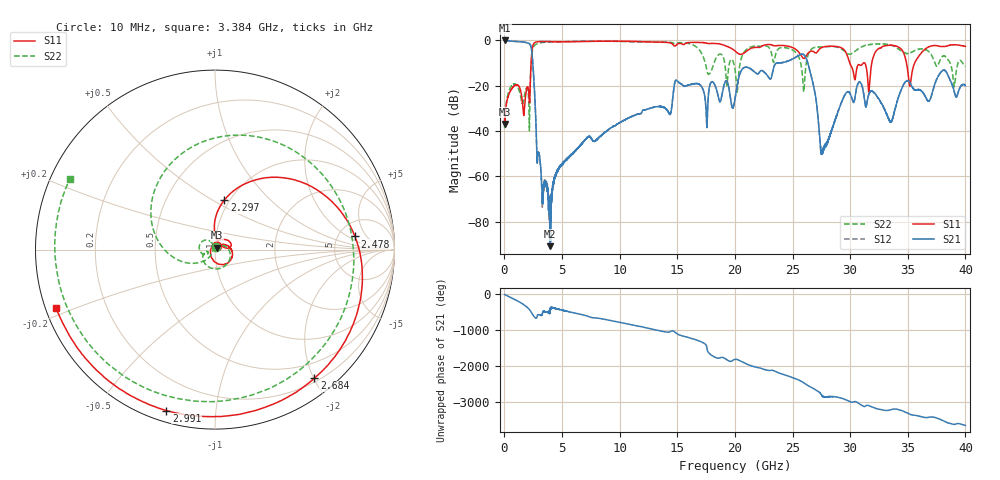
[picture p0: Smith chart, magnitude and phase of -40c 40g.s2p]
!Keysight Technologies,N5234A,MY52241180,A.10.60.03
!Date: Thursday, February 22, 2024 12:18:21
!Correction: S11(Full 2 Port(1,2))
!S21(Full 2 Port(1,2))
!S12(Full 2 Port(1,2))
!S22(Full 2 Port(1,2))
!S2P File: Measurements: S11, S21, S12, S22:
# Hz S  dB  R 50
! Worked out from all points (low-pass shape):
!   6401 points, 10 MHz to 40 GHz, reference 50 ohm
!   highest |S21| = -0.07 dB at 16.25 MHz (marker M1); lowest = -90.8 dB at 3.953 GHz (marker M2)
!   |S21| within 3 dB of the highest: start of sweep to 2.309 GHz
!   lowest |S11| = -36.9 dB at 16.25 MHz (marker M3), VSWR 1.03, Z = 51 + j1.05 ohm
!   |S11| at or under -10 dB: start of sweep to 2.308 GHz; 29.96 GHz to 31.15 GHz (1.188 GHz wide, 3.89 % of centre); 34.89 GHz to 35.59 GHz (706.8 MHz wide, 2.01 % of centre)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
!   |S22| runs from -39.9 to -0.4 dB; largest |S21 - S12| = 0.0083
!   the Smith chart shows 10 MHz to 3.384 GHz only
!   S11 on the Smith chart (normalised r, x): 10 MHz: 1.02, +0.04; 2.297 GHz: 0.95, +0.57; 2.478 GHz: 7.18, +2.71; 2.684 GHz: 0.25, -2.01; 2.991 GHz: 0.05, -0.74; 3.384 GHz: 0.03, -0.18
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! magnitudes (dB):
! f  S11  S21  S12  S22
! 10 MHz  -33.1  -0.1  -0.1  -36.2
! 16.25 MHz  -36.9  -0.1  -0.1  -39.3
! 1.703 GHz  -32.3  -0.8  -0.8  -25.2
! 2.297 GHz  -11.0  -2.8  -2.8  -11.6
! 2.478 GHz  -2.1  -11.6  -11.6  -3.4
! 2.684 GHz  -0.9  -30.7  -30.7  -1.9
! 2.991 GHz  -0.6  -49.7  -49.7  -1.2
! 3.384 GHz  -0.5  -65.5  -66.4  -0.9
! 3.953 GHz  -0.6  -90.8  -80.6  -0.8
! 6.677 GHz  -0.5  -45.9  -45.7  -0.4
! 13.34 GHz  -0.8  -29.2  -29.2  -0.8
! 14.97 GHz  -1.8  -17.8  -17.8  -1.2
! 20 GHz  -4.7  -25.9  -25.8  -12.8
! 20.88 GHz  -5.3  -11.9  -11.9  -4.6
! 24.9 GHz  -3.0  -8.4  -8.5  -4.0
! 25.95 GHz  -8.0  -6.3  -6.3  -22.2
! 26.67 GHz  -4.8  -16.8  -16.7  -3.7
! 27.6 GHz  -3.1  -48.3  -48.5  -2.9
! 30.78 GHz  -10.7  -18.5  -18.5  -3.6
! 33.34 GHz  -2.2  -34.7  -34.7  -1.9
! 35.19 GHz  -20.1  -18.7  -18.7  -5.6
! 40 GHz  -2.7  -20.0  -20.0  -11.5
